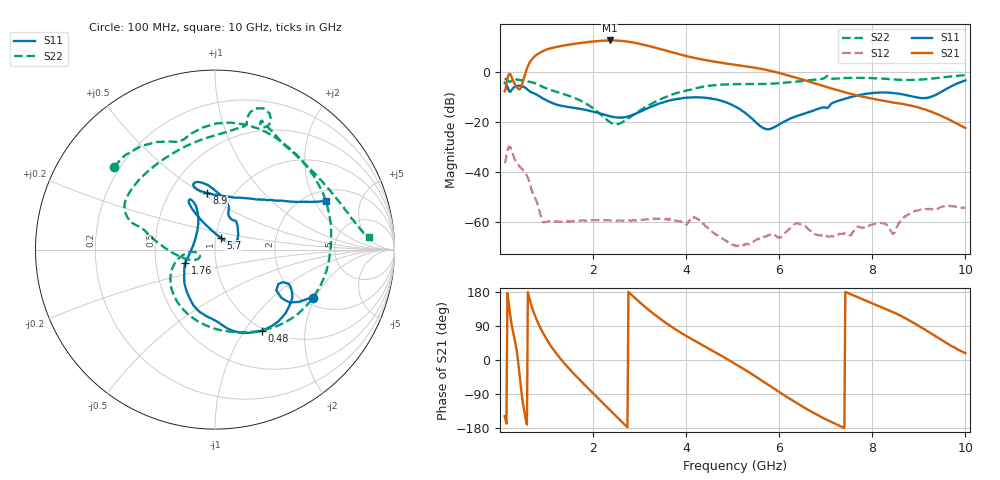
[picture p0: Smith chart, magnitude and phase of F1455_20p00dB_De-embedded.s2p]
! Integrated Device Technology
! Corporate Headquarters
! 6024 Silver Creek Valley Road
! San Jose, CA 95138  USA
! Phone:  1-408-284-8200
! Toll Free:  1-800-223-1366
! Webpage:  http://www.idt.com/
! Timing and RF Division
! 515 Groton Road, Suite 102
! Westford, MA 01886-6024
! Device:  F1455
! Description: 6-bit 0.5 dB Transmit Variable Gain Amplifier
! Frequency:  1400.0 -  2300.00 MHz
! Package:  6x6 mm Thin QFN Plastic Package: 28 pin
! State:  40
! Atten State:  20.0 dB
! Voltage:  +5.00 Volts
! Current:  217.627 mA
! Data:  The device was measured on a the F1455 evaluation board which has
!  individual transmission lines to the RF pins.  Data was collected
!  using a calibrated network analyzer.  The evaluation board was
!  de-embedded using a TRL calibration technique.
!  The reference plane is the edge of the package pin.
!  Pin  1 = CSb
!  Pin  2 = DATA
!  Pin  3 = CLK
!  Pin  4 = RSET
!  Pin  5 = GND
!  Pin  6 = RFIN  = Port 1
!  Pin  7 = GND
!  Pin  8 = NC
!  Pin  9 = NC
!  Pin 10 = NC
!  Pin 11 = NC
!  Pin 12 = NC
!  Pin 13 = NC
!  Pin 14 = /STBY
!  Pin 15 = GND
!  Pin 16 = RFOUT  = Port 2
!  Pin 17 = GND
!  Pin 18 = NC
!  Pin 19 = NC
!  Pin 20 = NC
!  Pin 21 = GND
!  Pin 22 = NC
!  Pin 23 = GND
!  Pin 24 = NC
!  Pin 25 = NC
!  Pin 26 = NC
!  Pin 27 = GND
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# GHz S dB R 50
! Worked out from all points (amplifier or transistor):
!   496 points, 100 MHz to 10 GHz, reference 50 ohm
!   highest |S21| = 12.6 dB at 2.36 GHz (marker M1)
!   |S21| within 3 dB of that: 1.117 GHz to 3.36 GHz (2.243 GHz wide, 100 % of centre)
!   unconditionally stable (mu >= 1): start of sweep to end of sweep
!   at 1.74 GHz: K = 108.26, MAG = 12.1 dB, |S12| = -59.3 dB
!   at 5.06 GHz: K = 685.72, MAG = 4.8 dB, |S12| = -69.4 dB
!   at 10 GHz: K = 465.72, MAG = -13.7 dB, |S12| = -54.3 dB
!   S11 on the Smith chart (normalised r, x): 100 MHz: 2.26, -1.93; 480 MHz: 0.97, -1.20; 1.76 GHz: 0.71, -0.11; 5.7 GHz: 1.05, +0.14; 8.9 GHz: 0.75, +0.53; 10 GHz: 2.47, +2.49
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0.1  -4.32 -26.2  -7.70 -148.4  -36.34 47.1  -2.76 140.7
0.26  -6.92 -24.8  -2.44 87.0  -31.85 -76.9  -3.31 95.8
0.38  -5.53 -41.9  -6.45 6.2  -36.78 -117.2  -3.04 57.8
0.48  -5.66 -60.2  -4.61 -101.8  -38.85 -148.5  -3.34 31.6
0.68  -8.12 -90.6  4.93 142.4  -47.05 139.9  -4.06 -15.1
0.82  -9.36 -108.8  7.29 97.2  -53.44 113.4  -5.00 -46.2
0.96  -10.94 -123.4  8.67 63.8  -59.96 126.1  -6.27 -71.5
1.34  -13.54 -144.5  10.47 -2.5  -59.72 98.1  -8.63 -121.1
1.76  -14.81 -155.7  11.66 -58.2  -59.28 65.7  -11.67 -156.0
2.06  -16.07 -163.9  12.30 -94.9  -59.20 49.6  -15.29 -171.5
2.36  -17.62 180.0  12.59 -131.7  -59.26 37.9  -19.95 -169.6
2.58  -18.20 161.0  12.46 -158.6  -59.26 30.4  -20.53 -154.1
2.78  -17.61 142.2  12.04 177.4  -59.24 25.6  -18.26 -152.3
3.08  -15.28 122.7  10.92 144.0  -59.01 18.3  -14.53 -166.3
3.4  -12.74 114.9  9.39 112.5  -58.48 7.2  -11.35 179.0
4.08  -10.16 116.0  6.02 57.9  -59.05 -5.4  -7.12 163.0
5.06  -13.80 116.9  2.88 -10.5  -69.44 -24.3  -4.84 148.0
5.7  -22.68 64.8  0.92 -60.2  -65.62 0.6  -4.76 121.9
6.7  -15.64 39.4  -4.15 -136.9  -63.70 -129.4  -3.18 78.4
8.36  -8.24 107.8  -11.95 130.5  -62.16 100.4  -2.82 62.4
8.9  -9.95 98.4  -13.77 97.4  -55.62 118.7  -3.16 40.9
10  -3.38 23.8  -22.33 18.2  -54.25 39.7  -1.28 4.6
